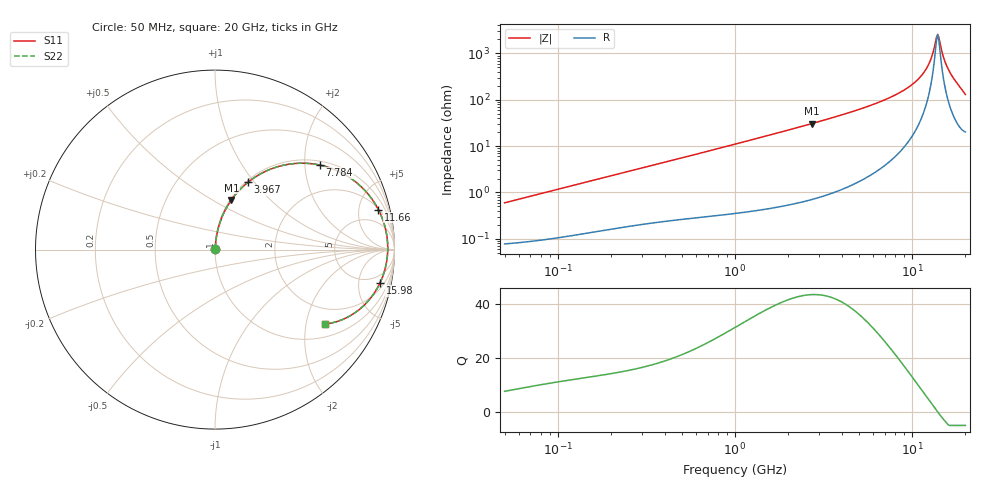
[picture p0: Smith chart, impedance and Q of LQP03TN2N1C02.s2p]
!Murata Part Number: LQP03TN2N1C02
!These Parameters are Measured in Series Mode Connection
!  o--[Z]--o
!Port1  Port2
!  o-------o
!Freq. Start=50[MHz] Stop=20[GHz], 401[Steps]
# Hz S RI R 50
!Freq.(Hz) S11(Real) S11(Imag) S21(Real) S21(Imag) S12(Real) S12(Imag) S22(Real) S22(Imag)
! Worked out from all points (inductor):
!   401 points, 50 MHz to 20 GHz, reference 50 ohm
!   read as one part in series: L = 1.88 nH near 51.52 MHz
!   highest Q = 43.4 at 2.728 GHz (marker M1), where L = 1.79 nH
!   self-resonance near 13.75 GHz
!   S11 on the Smith chart (normalised r, x): 50 MHz: 1.00, +0.01; 3.967 GHz: 1.02, +0.93; 7.784 GHz: 1.11, +2.39; 11.66 GHz: 2.10, +7.71; 15.98 GHz: 2.93, -9.04; 20 GHz: 1.40, -2.57
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5e7  0.00081 0.00592  0.9992 -0.00592  0.9992 -0.00592  0.00081 0.00592
1.364002e8  0.00151 0.0158  0.9985 -0.0158  0.9985 -0.0158  0.00151 0.0158
3.721004e8  0.004 0.0414  0.996 -0.0414  0.996 -0.0414  0.004 0.0414
1e9  0.0153 0.108  0.9847 -0.108  0.9847 -0.108  0.0153 0.108
2.728004e9  0.0916 0.2772  0.9084 -0.2772  0.9084 -0.2772  0.0916 0.2772
3.967106e9  0.184 0.3755  0.816 -0.3755  0.816 -0.3755  0.184 0.3755
5.433528e9  0.3251 0.4539  0.6749 -0.4539  0.6749 -0.4539  0.3251 0.4539
7.442007e9  0.5463 0.4775  0.4537 -0.4775  0.4537 -0.4775  0.5463 0.4775
7.784049e9  0.584 0.4711  0.416 -0.4711  0.416 -0.4711  0.584 0.4711
9.892087e9  0.792 0.3703  0.208 -0.3703  0.208 -0.3703  0.792 0.3703
1.082228e10  0.862 0.2982  0.138 -0.2982  0.138 -0.2982  0.862 0.2982
1.166392e10  0.91 0.2233  0.09 -0.2233  0.09 -0.2233  0.91 0.2233
1.257102e10  0.9445 0.1363  0.0555 -0.1363  0.0555 -0.1363  0.9445 0.1363
1.295331e10  0.9536 0.0987  0.0464 -0.0987  0.0464 -0.0987  0.9536 0.0987
1.354865e10  0.9614 0.0398  0.0386 -0.0398  0.0386 -0.0398  0.9614 0.0398
1.375312e10  0.9624 0.0197  0.0376 -0.0197  0.0376 -0.0197  0.9624 0.0197
1.396067e10  0.9624 -0.000648  0.0376 0.000648  0.0376 0.000648  0.9624 -0.000648
1.417136e10  0.9616 -0.0211  0.0384 0.0211  0.0384 0.0211  0.9616 -0.0211
1.504638e10  0.9487 -0.104  0.0513 0.104  0.0513 0.104  0.9487 -0.104
1.597544e10  0.9192 -0.1861  0.0808 0.1861  0.0808 0.1861  0.9192 -0.1861
1.774144e10  0.8218 -0.3185  0.1782 0.3185  0.1782 0.3185  0.8218 -0.3185
2e10  0.6116 -0.4152  0.3884 0.4152  0.3884 0.4152  0.6116 -0.4152
